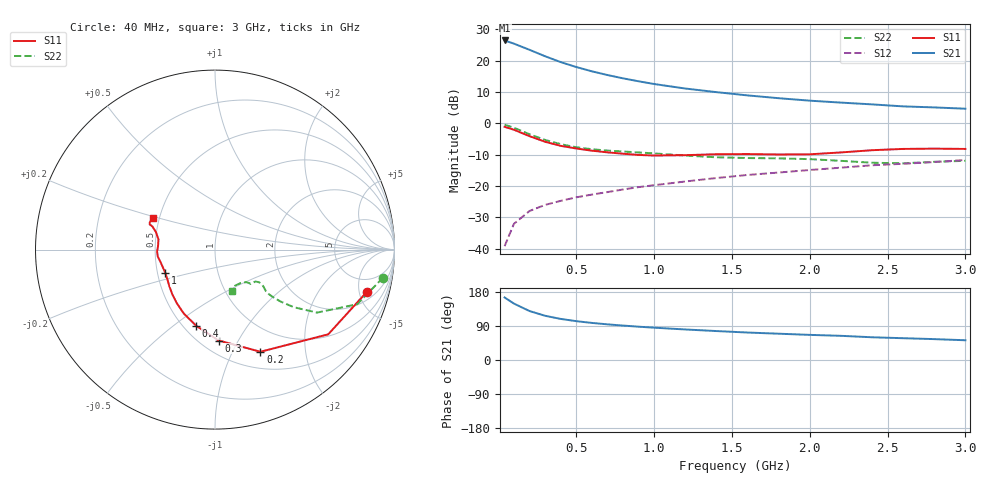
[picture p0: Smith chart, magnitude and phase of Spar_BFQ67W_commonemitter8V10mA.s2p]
! Filename:  BFQ67WI.S2P  Version:  4.0
! NXP part #: BFQ67W  Date: Jun 1994
! Bias condition: Vce=8V, Ic=10mA
#  MHz  S  MA  R  50
! Freq  S11  S21  S12  S22  !GUM [dB]
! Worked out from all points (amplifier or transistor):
!   21 points, 40 MHz to 3 GHz, reference 50 ohm
!   highest |S21| = 26.4 dB at 40 MHz (marker M1)
!   |S21| within 3 dB of that: start of sweep to 200.9 MHz
!   unconditionally stable (mu >= 1): 863.3 MHz to end of sweep
!   at 300 MHz: K = 0.61, MSG = 23.7 dB, |S12| = -26.0 dB
!   at 1 GHz: K = 1.05, MAG = 14.8 dB, |S12| = -19.7 dB
!   at 3 GHz: K = 1.04, MAG = 7.0 dB, |S12| = -11.7 dB
!   lowest NFmin = 1.80 dB at 1 GHz
!   S11 on the Smith chart (normalised r, x): 40 MHz: 2.87, -5.89; 200 MHz: 0.69, -1.29; 300 MHz: 0.61, -0.83; 400 MHz: 0.58, -0.61; 1 GHz: 0.55, -0.16; 3 GHz: 0.46, +0.19
40  0.877 -15.7  20.87 165.0  0.011 80.1  0.949 -9.5
100  0.788 -36.8  18.56 148.8  0.025 69.8  0.849 -21.0
200  0.623 -66.0  14.81 129.2  0.04 60.4  0.668 -31.7
300  0.507 -87.7  11.7 116.7  0.05 57.3  0.543 -36.2
400  0.437 -103.9  9.441 108.4  0.058 57.6  0.465 -38.4
500  0.396 -116.1  7.877 102.5  0.066 58.4  0.415 -39.4
600  0.366 -125.7  6.734 97.9  0.073 59.8  0.386 -39.6
700  0.344 -133.8  5.874 94.1  0.08 61.4  0.367 -39.3
800  0.327 -140.9  5.205 90.9  0.088 62.9  0.355 -38.5
900  0.313 -147.9  4.668 87.9  0.096 64.0  0.343 -37.6
1000  0.306 -154.6  4.224 85.3  0.103 64.9  0.331 -36.8
1200  0.31 -165.8  3.58 80.6  0.118 66.4  0.306 -36.5
1400  0.321 -173.0  3.134 76.4  0.134 67.7  0.287 -38.3
1600  0.323 -178.1  2.781 72.5  0.15 67.8  0.279 -41.8
1800  0.318 176.7  2.509 69.4  0.164 68.7  0.276 -43.8
2000  0.32 169.8  2.292 66.3  0.18 69.3  0.268 -44.4
2200  0.343 163.5  2.135 63.8  0.196 70.0  0.252 -46.0
2400  0.372 159.7  2 60.0  0.214 69.8  0.235 -52.4
2600  0.39 158.9  1.858 57.5  0.226 69.3  0.23 -60.6
2800  0.394 157.3  1.789 55.1  0.241 69.8  0.243 -65.4
3000  0.39 153.2  1.706 52.1  0.26 69.6  0.252 -67.6
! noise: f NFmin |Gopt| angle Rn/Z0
1000  1.8  0.363  70  0.253
